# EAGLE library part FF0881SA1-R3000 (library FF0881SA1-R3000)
FFC & FPC Connectors 81P 0.2MM FPC Source: Datasheet
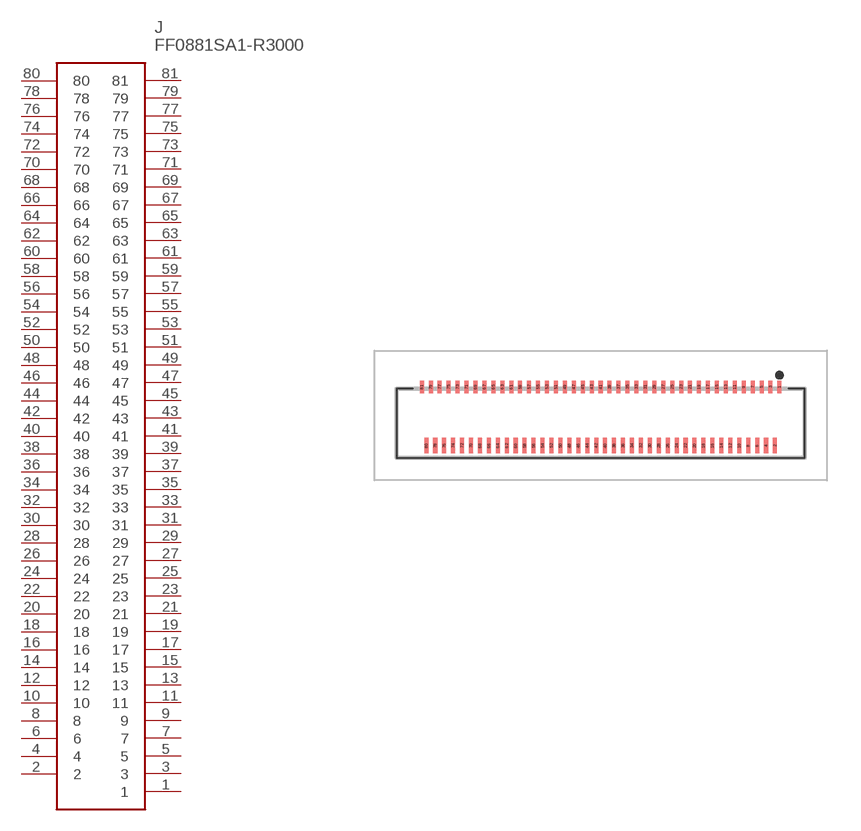
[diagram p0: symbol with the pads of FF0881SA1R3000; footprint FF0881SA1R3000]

Designator prefix J

## FF0881SA1-R3000 (Description: FFC & FPC Connectors 81P 0.2MM FPC; Height: 1mm; Manufacturer_Name: JAE Electronics; Manufacturer_Part_Number: FF0881SA1-R3000; Mouser_Part_Number: 656-FF0881SA1-R3000; Mouser_Price-Stock: https://www.mouser.co.uk/ProductDetail/JAE-Electronics/FF0881SA1-R3000?qs=e3doH35UsB4mcpzu8vQ7Tw%3D%3D)  [FF0881SA1R3000]
1  1
2  2
3  3
4  4
5  5
6  6
7  7
8  8
9  9
10  10
11  11
12  12
13  13
14  14
15  15
16  16
17  17
18  18
19  19
20  20
21  21
22  22
23  23
24  24
25  25
26  26
27  27
28  28
29  29
30  30
31  31
32  32
33  33
34  34
35  35
36  36
37  37
38  38
39  39
40  40
41  41
42  42
43  43
44  44
45  45
46  46
47  47
48  48
49  49
50  50
51  51
52  52
53  53
54  54
55  55
56  56
57  57
58  58
59  59
60  60
61  61
62  62
63  63
64  64
65  65
66  66
67  67
68  68
69  69
70  70
71  71
72  72
73  73
74  74
75  75
76  76
77  77
78  78
79  79
80  80
81  81

## Footprint FF0881SA1R3000 (pad centres in mm)
FF0881SA1-R3000
smd 0.18 x 0.55: 1 8,1.274; 3 7.6,1.274; 5 7.2,1.274; 7 6.8,1.274; 9 6.4,1.274; 11 6,1.274; 13 5.6,1.274; 15 5.2,1.274; 17 4.8,1.274; 19 4.4,1.274; 21 4,1.274; 23 3.6,1.274; 25 3.2,1.274; 27 2.8,1.274; 29 2.4,1.274; 31 2,1.274; 33 1.6,1.274; 35 1.2,1.274; 37 0.8,1.274; 39 0.4,1.274; 41 0,1.274; 43 -0.4,1.274; 45 -0.8,1.274; 47 -1.2,1.274; 49 -1.6,1.274; 51 -2,1.274; 53 -2.4,1.274; 55 -2.8,1.274; 57 -3.2,1.274; 59 -3.6,1.274; 61 -4,1.274; 63 -4.4,1.274; 65 -4.8,1.274; 67 -5.2,1.274; 69 -5.6,1.274; 71 -6,1.274; 73 -6.4,1.274; 75 -6.8,1.274; 77 -7.2,1.274; 79 -7.6,1.274; 81 -8,1.274
smd 0.18 x 0.7: 2 7.8,-1.351; 4 7.4,-1.351; 6 7,-1.351; 8 6.6,-1.351; 10 6.2,-1.351; 12 5.8,-1.351; 14 5.4,-1.351; 16 5,-1.351; 18 4.6,-1.351; 20 4.2,-1.351; 22 3.8,-1.351; 24 3.4,-1.351; 26 3,-1.351; 28 2.6,-1.351; 30 2.2,-1.351; 32 1.8,-1.351; 34 1.4,-1.351; 36 1,-1.351; 38 0.6,-1.351; 40 0.2,-1.351; 42 -0.2,-1.351; 44 -0.6,-1.351; 46 -1,-1.351; 48 -1.4,-1.351; 50 -1.8,-1.351; 52 -2.2,-1.351; 54 -2.6,-1.351; 56 -3,-1.351; 58 -3.4,-1.351; 60 -3.8,-1.351; 62 -4.2,-1.351; 64 -4.6,-1.351; 66 -5,-1.351; 68 -5.4,-1.351; 70 -5.8,-1.351; 72 -6.2,-1.351; 74 -6.6,-1.351; 76 -7,-1.351; 78 -7.4,-1.351; 80 -7.8,-1.351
